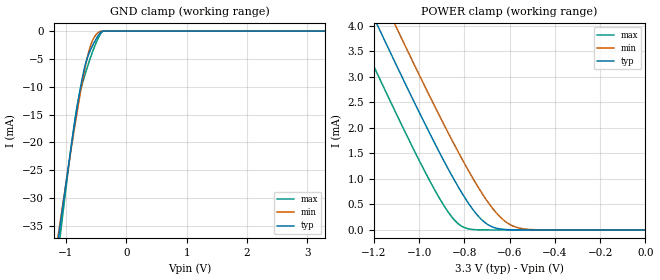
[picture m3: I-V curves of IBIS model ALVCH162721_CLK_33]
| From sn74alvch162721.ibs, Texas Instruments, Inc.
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[Model]   ALVCH162721_CLK_33
Model_type  Input
Vinl = 0.8
Vinh = 2.0
| variable   typ   min   max
C_comp   1.96pF   1.71pF   2.69pF
[Temperature Range]   40   100   -40
| Ambient temperature   25   85   -40
[Voltage range]   3.3   3   3.6
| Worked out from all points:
|   GND clamp passes 1 mA (typ) near -0.48 V on its own axis
|   POWER clamp passes 1 mA (typ) near -0.85 V on its own axis
[GND Clamp]
| ALVCH162721_CLK_33
|   Voltage   I(typ)   I(min)   I(max)
-3.3V     -222.4mA   -207.7mA   -245.4mA
-1.125V   -37.37mA   -36.52mA   -39.57mA
-1.095V   -34.97mA   -34.31mA   -36.86mA
-1.065V   -32.59mA   -32.11mA   -34.16mA
-855mV    -16.59mA   -17.25mA   -16.23mA
-790mV    -12.12mA   -12.96mA   -12.11mA
-720mV    -7.968mA   -8.671mA   -9.142mA
-660mV    -5.336mA   -5.456mA   -7.005mA
-585mV    -3.229mA   -2.435mA   -4.541mA
-440mV    -448uA     -97.75uA   -766.1uA
-375mV    -85.17nA   -8.524uA   -4.38uA
3.3V      45.43pA    164.4pA    42.9pA
[POWER Clamp]
| ALVCH162721_CLK_33
|   Voltage   I(typ)   I(min)   I(max)
-3.3V     24.83mA    25.52mA    23.96mA
-1.275V   4.872mA    5.61mA     3.918mA
-1.185V   4.018mA    4.758mA    3.062mA
-1.105V   3.269mA    4.008mA    2.314mA
-1.07V    2.945mA    3.683mA    1.992mA
-940mV    1.776mA    2.501mA    856.4uA
-845mV    982.9uA    1.676mA    200.1uA
-795mV    611.2uA    1.266mA    38.41uA
-725mV    207uA      738.7uA    1.527uA
-625mV    11.21uA    186.8uA    11.91nA
-510mV    181.6nA    9.688uA    52.91pA
-48.03fV  6.303pA    7.801pA    6.677pA
